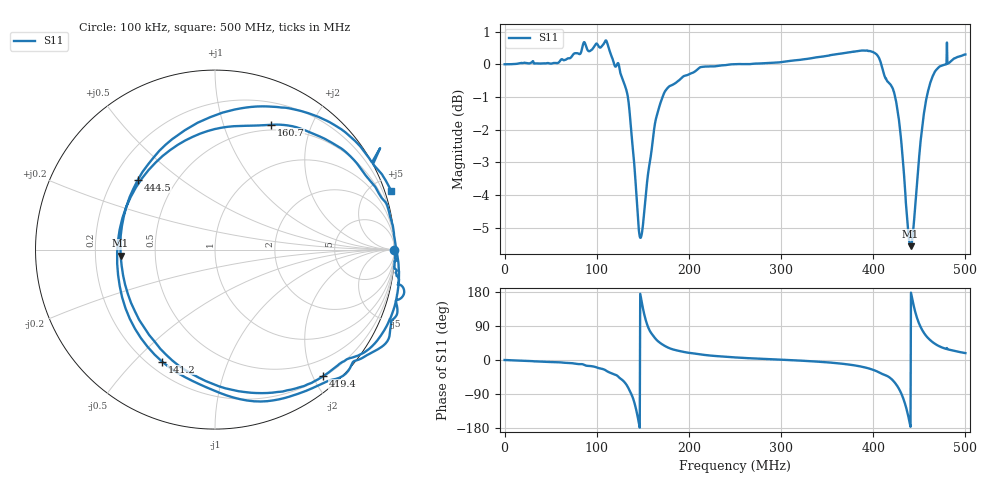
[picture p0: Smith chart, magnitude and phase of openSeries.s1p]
# Hz S RI R 50.0
! written by SimSmith version 18.3h
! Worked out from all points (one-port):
!   1000 points, 100 kHz to 500 MHz, reference 50 ohm
!   lowest |S11| = -5.6 dB at 440.5 MHz (marker M1), VSWR 3.23, Z = 15.5 - j1.46 ohm
!   |S11| at or under -10 dB: nowhere
!   S11 on the Smith chart (normalised r, x): 100 kHz: open; 141.2 MHz: 0.25, -0.60; 160.7 MHz: 0.44, +1.46; 419.4 MHz: 0.21, -2.16; 444.5 MHz: 0.30, +0.36; 500 MHz: -0.68, +6.16
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100000  1 -0.000149
6.265005e7  1.01 -0.1235
8.316647e7  1.026 -0.1947
1.081865e8  0.9753 -0.459
1.252001e8  0.6547 -0.7242
1.347077e8  0.2171 -0.8452
1.412129e8  -0.2947 -0.6244
1.447157e8  -0.5176 -0.2655
1.482185e8  -0.516 0.1748
1.537229e8  -0.1237 0.6285
1.607285e8  0.3134 0.6962
1.722377e8  0.6915 0.5713
1.877502e8  0.8544 0.3951
2.503002e8  0.9933 0.1182
3.128503e8  1.013 -0.0116
3.754003e8  1.019 -0.2276
4.009207e8  0.9299 -0.4706
4.194355e8  0.6045 -0.7043
4.299439e8  0.057 -0.7726
4.339471e8  -0.238 -0.6176
4.379504e8  -0.4674 -0.2977
4.404524e8  -0.5259 -0.034
4.444556e8  -0.4291 0.3902
4.484588e8  -0.1678 0.6652
4.52462e8  0.1083 0.7802
4.654724e8  0.6792 0.6857
4.77482e8  0.86 0.5077
5e8  0.9832 0.3238
